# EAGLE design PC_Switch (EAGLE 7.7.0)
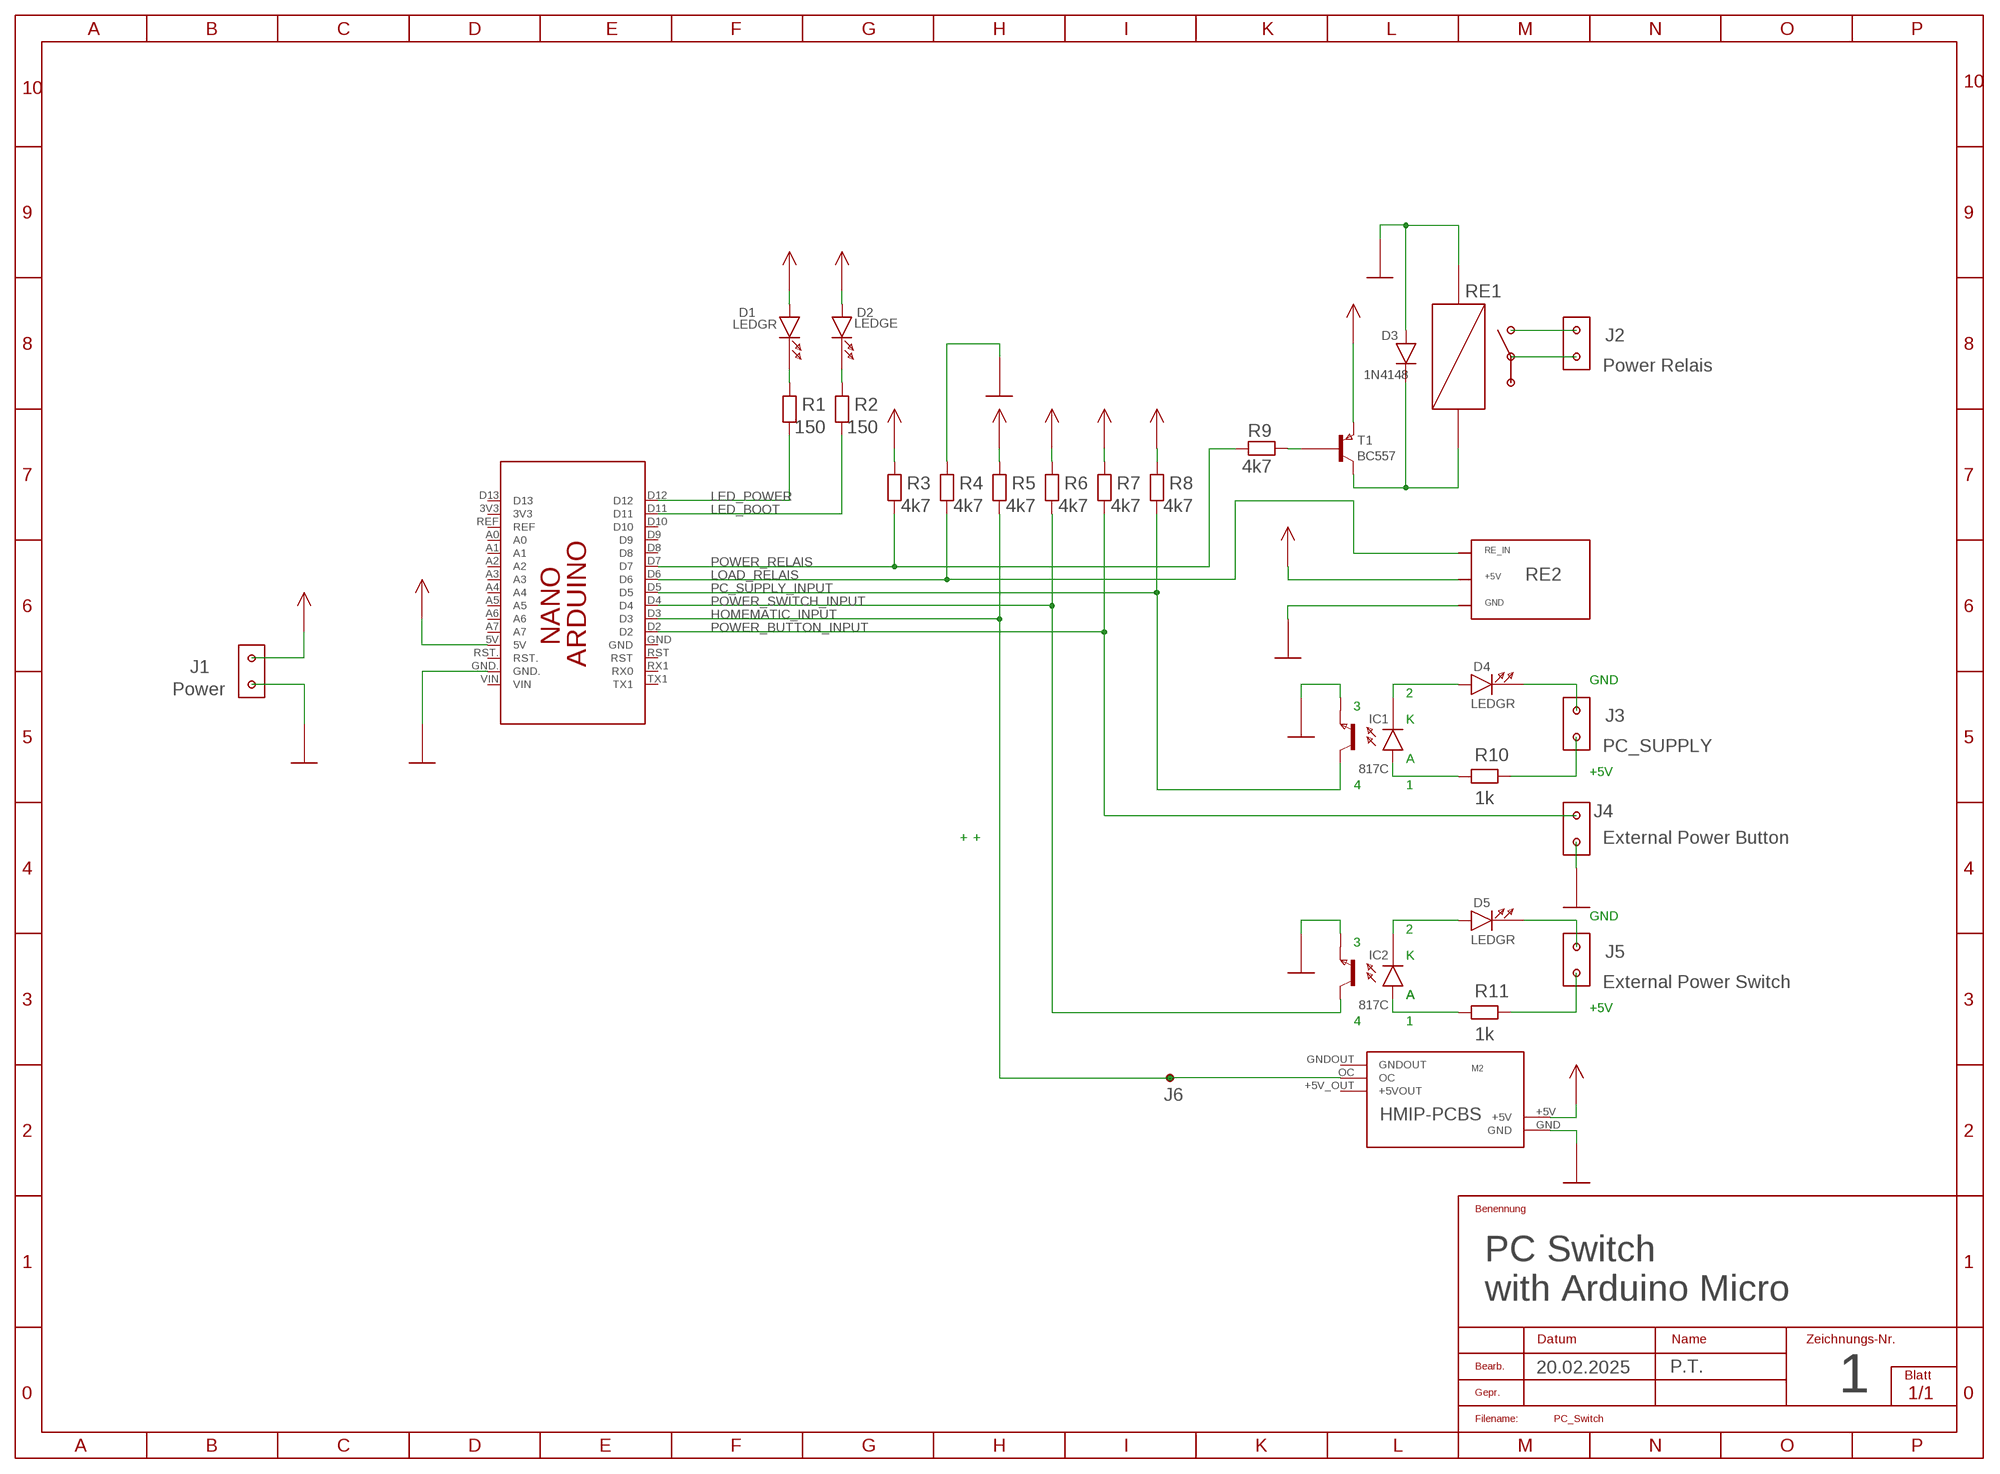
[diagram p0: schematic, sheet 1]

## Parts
D1  LEDGR  LED5GR  [LED5SGR]
D2  LEDGE  LED5GE  [LED5SGE]
D3  1N4148  [DIODE03B]
D4  LEDGR  LED3ROT  [LED3SROT]
D5  LEDGR  LED3ROT  [LED3SROT]
IC1  817C  [DIL4]
IC2  817C  [DIL4]
J1  Power  POWER2X1  [POWER2X1]
J2  Power Relais  POWER2X1  [POWER2X1]
J3  PC_SUPPLY  POWER2X1  [POWER2X1]
J4  External Power Button  POWER2X1  [POWER2X1]
J5  External Power Switch  POWER2X1  [POWER2X1]
J6  PIN  [PIN]
M2  HMIP_PCBS  [HMIP_PCBS]
PCB1  ARDUINO_NANO_PT  [ARDUINO_NANO_PT]
R1  150  RES04  [RES04B]
R2  150  RES04  [RES04B]
R3  4k7  RES04  [RES04B]
R4  4k7  RES06H  [RES06B1]
R5  4k7  RES03H  [RES03B1]
R6  4k7  RES04H  [RES04B1]
R7  4k7  RES02  [RES02B]
R8  4k7  RES05H  [RES05B1]
R9  4k7  RES04  [RES04B]
R10  1k  RES04  [RES04B]
R11  1k  RES04  [RES04B]
RE1  REL_ELV  [REL_ELV]
RE2  RE3  REL_MOD1  [REL_MOD1]
T1  BC557  [TO92A]

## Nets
GND: D3.A IC1.3(E) IC2.3(E) J1.2 J4.1 M2.GND PCB1.GND. R4.2 RE1.SP1 RE2.GND
HOMEMATIC_INPUT: J6.1 M2.OC PCB1.D3 R5.1
LED_BOOT: PCB1.D11 R2.1
LED_POWER: PCB1.D12 R1.1
LOAD_RELAIS: PCB1.D6 R4.1 RE2.RE_IN
N$1: D5.A IC2.2(K)
N$2: IC2.1(A) R11.1
N$3: D4.K J3.2
N$4: D1.K R1.2
N$5: D2.K R2.2
N$6: R9.2 T1.2(B)
N$7: D5.K J5.2
N$8: J5.1 R11.2
N$9: J3.1 R10.2
N$10: D3.K RE1.SP2 T1.1(C)
N$11: D4.A IC1.2(K)
N$12: J2.1 RE1.COM1(COM) RE1.COM2(COM)
N$13: J2.2 RE1.NO
N$14: IC1.1(A) R10.1
PC_SUPPLY_INPUT: IC1.4(C) PCB1.D5 R8.1
POWER_BUTTON_INPUT: J4.2 PCB1.D2 R7.1
POWER_RELAIS: PCB1.D7 R3.1 R9.1
POWER_SWITCH_INPUT: IC2.4(C) PCB1.D4 R6.1
VCC: D1.A D2.A J1.1 M2.+5V PCB1.5V R3.2 R5.2 R6.2 R7.2 R8.2 RE2.+5V T1.3(E)
Unconnected: PCB1.3V3 PCB1.A0 PCB1.A1 PCB1.A2 PCB1.A3 PCB1.A4 PCB1.A5 PCB1.A6 PCB1.A7 PCB1.D8 PCB1.D9 PCB1.D10 PCB1.D13 PCB1.GND PCB1.REF PCB1.RST PCB1.RST. PCB1.RX1(RX0) PCB1.TX1 PCB1.VIN RE1.NC

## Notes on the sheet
- GND
- 2
- 3
- K
- A
- +5V
- 4 | 1
- + | +
- GND
- 2
- 3
- K
- A | A
- +5V
- 4 | 1
- PC Switch
- with Arduino Micro
- 20.02.2025 | P.T.
- 1

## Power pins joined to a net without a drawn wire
+5VOUT: M2.+5V_OUT(+5VOUT)
GNDOUT: M2.GNDOUT

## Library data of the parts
D1 = Opto:LED5GR
D2 = Opto:LED5GE
D3 = Diode Triac:1N4148
D4 D5 = Opto:LED3ROT
IC1 IC2 = Opto:817C
J1-J5 = Connector 2:POWER2X1
J6 = Connector 2:PIN
M2 = Giess:HMIP_PCBS
PCB1 = Arduino:ARDUINO_NANO_PT: Device for representing an Arduino Nano board with a footprint in an EAGLE design. Created by Dave Young for Element14. More EAGLE documentation at: http://www.element14.com/community/community/knode/cadsoft_eagle
R1-R3 R9-R11 = Discrete:RES04
R4 = Discrete:RES06H
R5 = Discrete:RES03H
R6 = Discrete:RES04H
R7 = Discrete:RES02
R8 = Discrete:RES05H
RE1 = Mechanic:REL_ELV
RE2 = Mechanic:REL_MOD1
T1 = Transistor:BC557

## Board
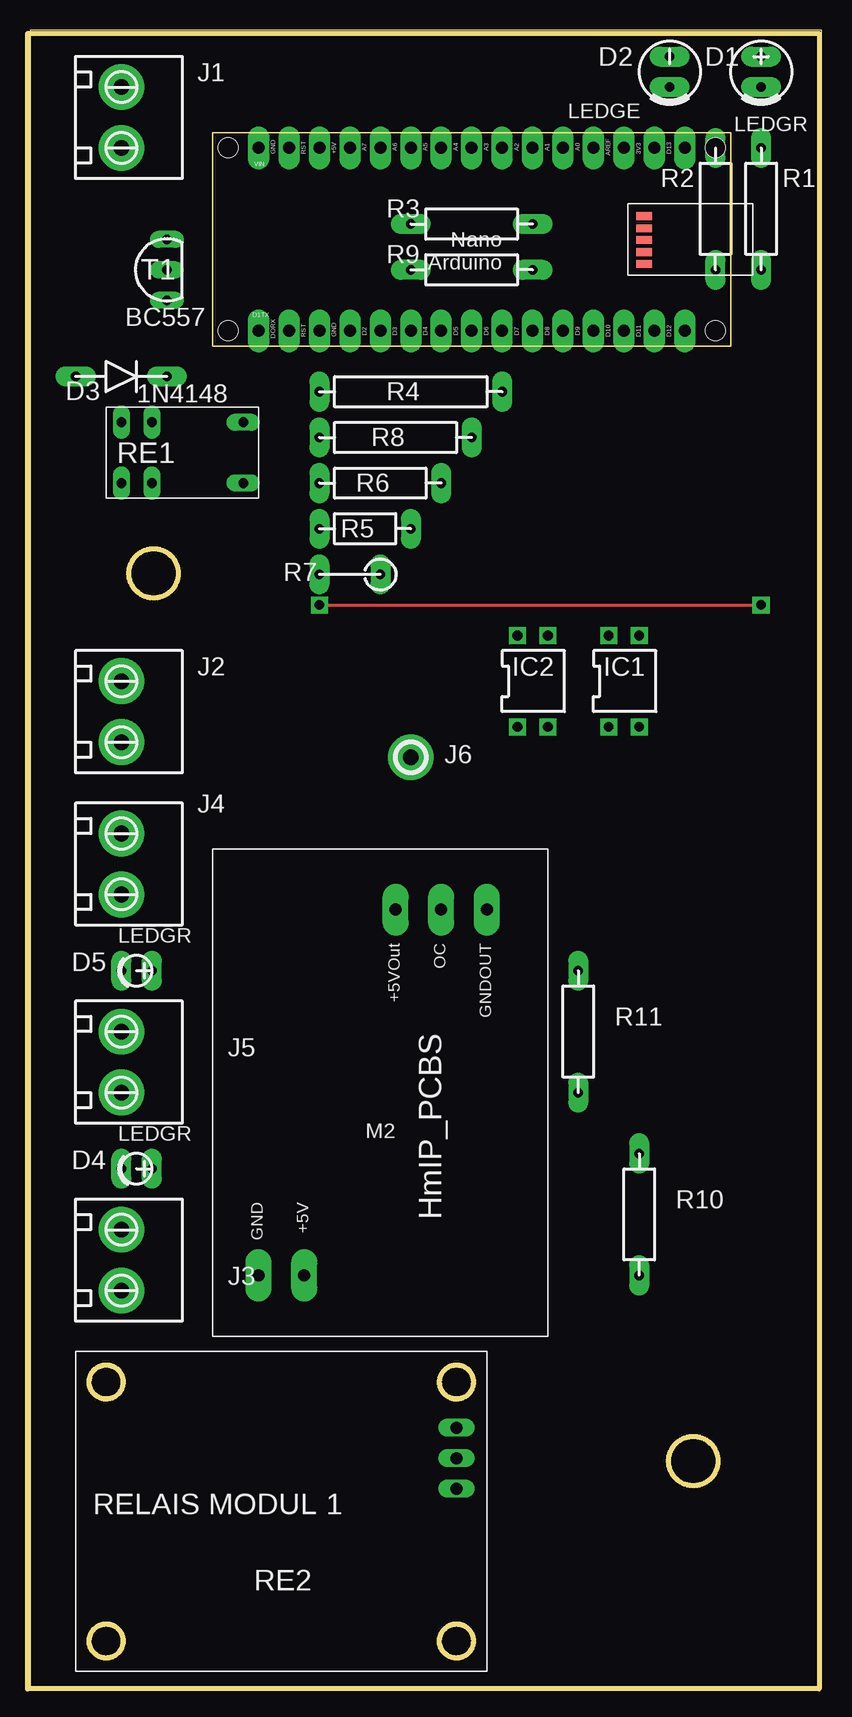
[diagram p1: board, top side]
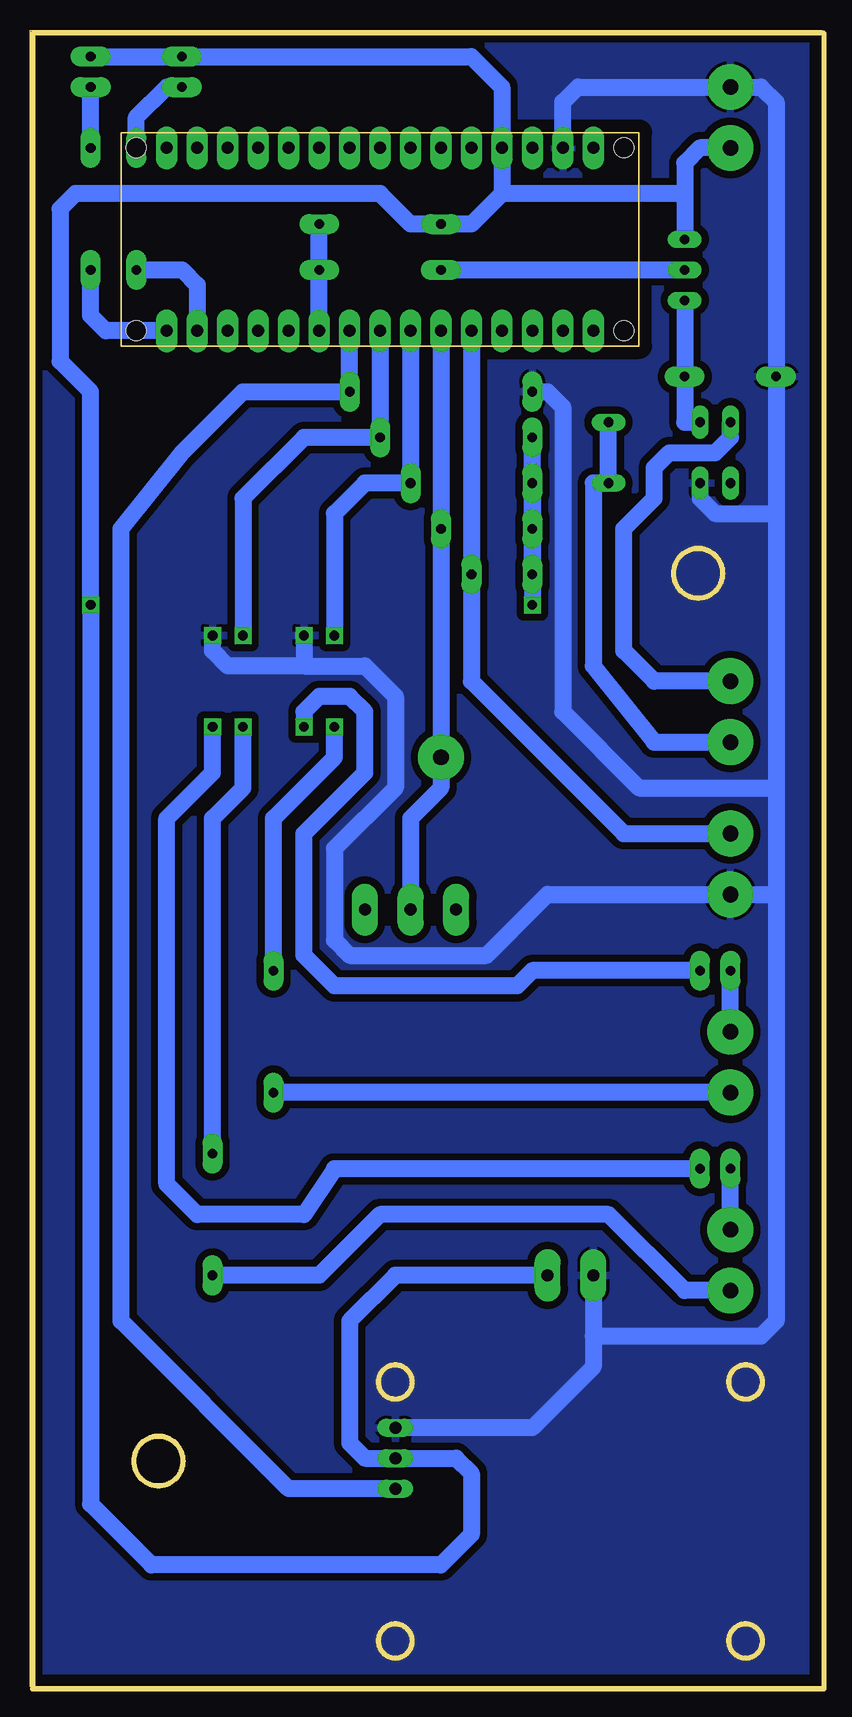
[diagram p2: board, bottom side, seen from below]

Size 66.02 x 138.1 mm. Coordinates in mm from the lower left corner, seen from the top.
Outline: 0,0 66.02,0 66.02,138.1 0,138.1 0,0
Copper layers (1*16): Top 0.035mm / dielectric 1.5mm / Bottom 0.035mm
Design rules "default": minimum track width 10mil, minimum drill 24mil, track to track 8mil, track to pad 8mil, pad to pad 8mil, via to via 8mil, smd to smd 8mil, copper to edge 40mil, drill to drill 8mil, minimum pad ring 10mil, minimum via ring 8mil, stop-mask expansion 4mil, vias tented up to drill 0mil, thermal gap 10mil
Milling: 20 lines

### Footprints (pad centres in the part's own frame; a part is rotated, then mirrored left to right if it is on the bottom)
LED5SGR = drill 0.8 pad 1.676 long: A 2.54,0; K 0,0
LED5SGE = drill 0.8 pad 1.676 long: A 2.54,0; K 0,0
DIODE03B = drill 0.8 pad 1.676 long: A 7.62,0; K 0,0
LED3SROT = drill 0.8 pad 1.676 long: A 2.54,0; K 0,0
DIL4 = drill 0.813 pad 1.422 square: 1 0,0; 2 2.54,0; 3 2.54,7.62; 4 0,7.62
POWER2X1 = drill 1.3 pad 3.81: 1 0,0; 2 0,5.08
PIN = drill 1.3 pad 3.81: 1 0,0
HMIP_PCBS = drill 1 pad 2.184 long: +5V 34.29,7.62; +5V_OUT 3.81,15.24; GND 34.29,3.81; GNDOUT 3.81,22.86; OC 3.81,19.05
ARDUINO_NANO_PT = drill 1 pad 1.778 long: 3V3 6.35,1.27; 5V 31.75,1.27; A0 11.43,1.27; A1 13.97,1.27; A2 16.51,1.27; A3 19.05,1.27; A4 21.59,1.27; A5 24.13,1.27; A6 26.67,1.27; A7 29.21,1.27; D2 29.21,16.51; D3 26.67,16.51; D4 24.13,16.51; D5 21.59,16.51; D6 19.05,16.51; D7 16.51,16.51; D8 13.97,16.51; D9 11.43,16.51; D10 8.89,16.51; D11 6.35,16.51; D12 3.81,16.51; D13 3.81,1.27; GND 31.75,16.51; GND. 36.83,1.27; REF 8.89,1.27; RST 34.29,16.51; RST. 34.29,1.27; RX1 36.83,16.51; TX1 39.37,16.51; VIN 39.37,1.27 | smd 1.27 x 0.635: <USB>+V 7.214,10.947; <USB>D+ 7.214,9.957; <USB>D- 7.214,8.941; <USB>GND 7.214,6.96; <USB>ID 7.214,7.976 | hole 1.651: 1.27,1.27; 1.27,16.51; 41.91,16.51; 41.91,1.27
RES04B = drill 0.8 pad 1.676 long: 1 0,0; 2 10.16,0
RES06B1 = drill 0.8 pad 1.676 long: 1 0,0; 2 15.24,0
RES03B1 = drill 0.8 pad 1.676 long: 1 0,0; 2 7.62,0
RES04B1 = drill 0.8 pad 1.676 long: 1 0,0; 2 10.16,0
RES02B = drill 0.8 pad 1.676 long: 1 0,0; 2 5.08,0
RES05B1 = drill 0.8 pad 1.676 long: 1 0,0; 2 12.7,0
REL_ELV = drill 0.8 pad 1.397 long: COM1 0,5.08; COM2 0,0; NC 10.16,5.08; NO 10.16,0; SP1 7.62,5.08; SP2 7.62,0
REL_MOD1 = drill 1 pad 1.397 long: +5V 2.54,8.89; GND 2.54,6.35; RE_IN 2.54,11.43
TO92A = drill 0.8 pad 1.422 long: 1 0,0; 2 2.54,0; 3 5.08,0

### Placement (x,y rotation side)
D1  60.96,133.35 90 top
D2  53.34,133.35 90 top
D3  11.43,109.22 180 top
D4  7.62,43.18 0 top
D5  7.62,59.69 0 top
IC1  48.26,80.01 0 top
IC2  40.64,80.01 0 top
J1  7.62,128.27 0 top
J2  7.62,78.74 0 top
J3  7.62,33.02 0 top
J4  7.62,66.04 0 top
J5  7.62,49.53 0 top
J6  31.75,77.47 0 top
M2  15.24,68.58 270 top
PCB1  58.42,129.54 180 top
R1  60.96,118.11 90 top
R2  57.15,118.11 90 top
R3  41.91,121.92 180 top
R4  39.37,107.95 180 top
R5  31.75,96.52 180 top
R6  34.29,100.33 180 top
R7  29.21,92.71 180 top
R8  36.83,104.14 180 top
R9  41.91,118.11 180 top
R10  50.8,44.45 270 top
R11  45.72,59.69 270 top
RE1  17.78,105.41 180 top
RE2  38.1,27.94 180 top
T1  11.43,115.57 90 top

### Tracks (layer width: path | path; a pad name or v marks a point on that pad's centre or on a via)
GND
  Bottom 1.422: PCB1.GND. 21.59,132.08 20.32,133.35 J1.2 5.08,133.35 3.81,132.08 D3.A 3.81,97.79 | RE1.SP1 10.16,99.06 8.89,97.79 3.81,97.79 | 3.81,97.79 3.81,74.93 | 3.81,74.93 3.81,66.04 | 3.81,66.04 J4.1 22.86,66.04 27.94,60.96 39.37,60.96 40.64,62.23 40.64,69.85 35.56,74.93 35.56,82.55 38.1,85.09 43.18,85.09 | 3.81,66.04 3.81,30.48 5.08,29.21 19.05,29.21 | M2.GND 19.05,29.21 | 19.05,29.21 19.05,26.67 24.13,21.59 RE2.GND | 43.18,85.09 49.53,85.09 50.8,86.36 IC1.3 | IC2.3 43.18,85.09 | R4.2 22.86,107.95 21.59,106.68 21.59,81.28 15.24,74.93 3.81,74.93
  pour Bottom (isolate 0.61): 1.27,137.16 64.77,137.16 66.04,135.89 66.04,1.27 64.77,0 1.27,0 0,1.27 0,135.89
HOMEMATIC_INPUT
  Bottom 1.422: PCB1.D3 R5.1 J6.1 31.75,74.93 34.29,72.39 M2.OC
LED_BOOT
  Bottom 1.422: R2.1 53.34,118.11 52.07,116.84 PCB1.D11
LED_POWER
  Bottom 1.422: PCB1.D12 59.69,113.03 60.96,114.3 R1.1
LOAD_RELAIS
  Bottom 1.422: PCB1.D6 R4.1 48.26,107.95 53.34,102.87 58.42,96.52 58.42,30.48 44.45,16.51 RE2.RE_IN
N$1
  Bottom 1.422: D5.A 24.13,59.69 25.4,58.42 40.64,58.42 43.18,60.96 43.18,71.12 38.1,76.2 38.1,81.28 39.37,82.55 41.91,82.55 43.18,81.28 IC2.2
N$2
  Bottom 1.422: R11.1 45.72,72.39 40.64,77.47 IC2.1
N$3
  Bottom 1.422: J3.2 D4.K
N$4
  Bottom 1.422: R1.2 D1.K
N$5
  Bottom 1.422: R2.2 57.15,130.81 54.61,133.35 D2.K
N$6
  Bottom 1.422: R9.2 T1.2
N$7
  Bottom 1.422: J5.2 D5.K
N$8
  Bottom 1.422: J5.1 R11.2
N$9
  Bottom 1.422: J3.1 11.43,33.02 17.78,39.37 36.83,39.37 41.91,34.29 R10.2
N$10
  Bottom 1.422: T1.1 D3.K 11.43,105.41 RE1.SP2
N$11
  Bottom 1.422: D4.A 40.64,43.18 43.18,39.37 52.07,39.37 54.61,41.91 54.61,72.39 50.8,76.2 IC1.2
N$12
  Bottom 1.422: RE1.COM2 RE1.COM1 19.05,100.33 19.05,85.09 13.97,78.74 J2.1
N$13
  Bottom 1.422: J2.2 13.97,83.82 16.51,86.36 16.51,96.52 13.97,99.06 13.97,101.6 12.7,102.87 8.89,102.87 7.62,104.14 RE1.NO
N$14
  Bottom 1.422: R10.1 50.8,72.39 48.26,74.93 IC1.1
PC_SUPPLY_INPUT
  Bottom 1.422: PCB1.D5 R8.1 43.18,104.14 48.26,99.06 IC1.4
POWER_BUTTON_INPUT
  Bottom 1.422: PCB1.D2 R7.1 29.21,83.82 16.51,71.12 J4.2
POWER_RELAIS
  Bottom 1.422: PCB1.D7 R9.1 R3.1
POWER_SWITCH_INPUT
  Bottom 1.422: PCB1.D4 R6.1 38.1,100.33 40.64,97.79 IC2.4
VCC  (via drill 0.8 pad 1.42)
  Top 0.254: v24.13,90.17 v60.96,90.17
  Bottom 1.422: D1.A D2.A 29.21,135.89 26.67,133.35 PCB1.5V 26.67,124.46 | 11.43,124.46 T1.3 | J1.1 10.16,128.27 11.43,127 11.43,124.46 | 11.43,124.46 26.67,124.46 | 26.67,124.46 29.21,121.92 R3.2 34.29,121.92 36.83,124.46 62.23,124.46 63.5,123.19 63.5,110.49 60.96,107.95 v60.96,90.17 60.96,15.24 55.88,10.16 31.75,10.16 29.21,12.7 29.21,17.78 30.48,19.05 RE2.+5V 38.1,19.05 39.37,20.32 39.37,30.48 35.56,34.29 M2.+5V | R5.2 R6.2 R7.2 | R7.2 R8.2 | R7.2 v24.13,90.17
